FUNCTION FC 61 : VOID
TITLE =Communication to next cell
//
VERSION : 0.1

BEGIN
NETWORK
TITLE =Loader Ready For Auto/Cycle
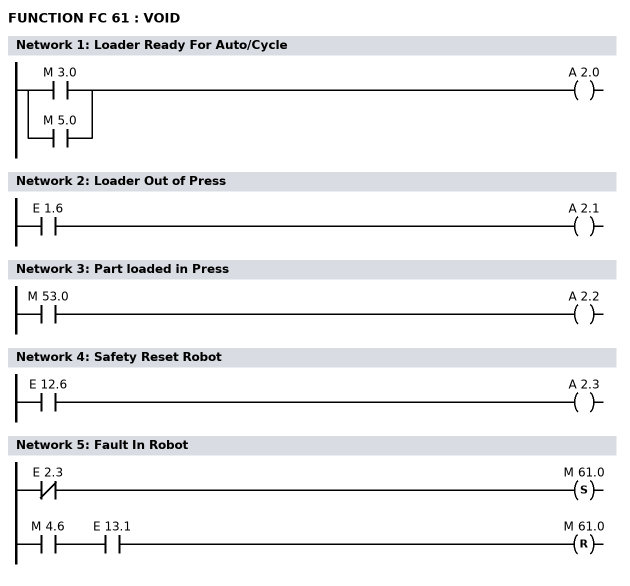
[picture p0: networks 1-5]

      O     M      3.0;
      O     M      5.0;
      =     A      2.0;
NETWORK
TITLE =Loader Out of Press

      U     E      1.6;
      =     A      2.1;
NETWORK
TITLE =Part loaded in Press

      U     M     53.0;
      =     A      2.2;
NETWORK
TITLE =Safety Reset Robot

      U     E     12.6;
      =     A      2.3;
NETWORK
TITLE =Fault In Robot

      UN    E      2.3;
      S     M     61.0;
      U     M      4.6;
      U     E     13.1;
      R     M     61.0;
      NOP   0;
END_FUNCTION

